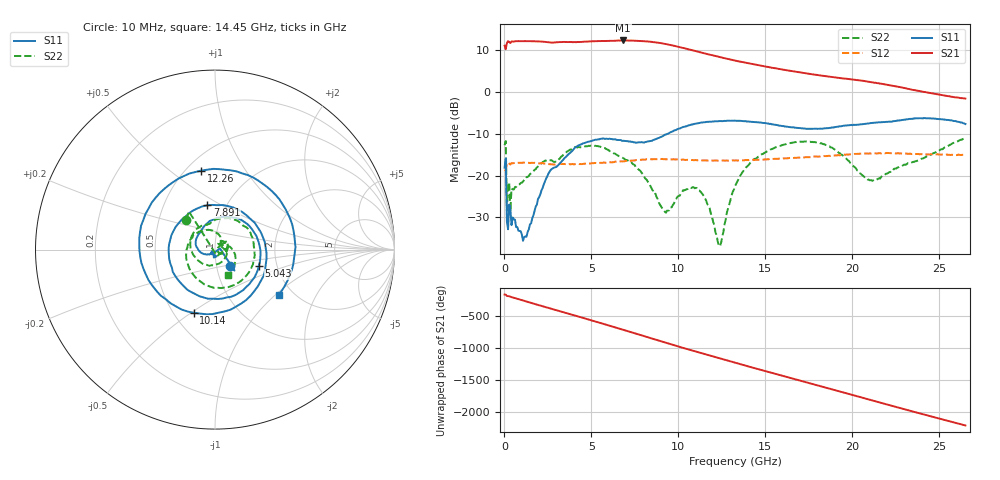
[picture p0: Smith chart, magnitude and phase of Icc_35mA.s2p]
!Keysight Technologies,N5245A,MY52451697,A.10.60.06
!Date: Thursday, May 06, 2021 15:08:13
!Correction: S11(Full 2 Port(1,4))
!S41(Full 2 Port(1,4))
!S14(Full 2 Port(1,4))
!S44(Full 2 Port(1,4))
!S2P File: Measurements: S11, S41, S14, S44:
# Hz S  dB  R 50
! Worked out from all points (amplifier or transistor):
!   401 points, 10 MHz to 26.5 GHz, reference 50 ohm
!   highest |S21| = 12.4 dB at 6.831 GHz (marker M1)
!   |S21| within 3 dB of that: start of sweep to 11.41 GHz
!   unconditionally stable (mu >= 1): start of sweep to end of sweep
!   at 4.381 GHz: K = 1.13, MAG = 12.4 dB, |S12| = -17.3 dB
!   at 13.26 GHz: K = 1.24, MAG = 9.0 dB, |S12| = -16.4 dB
!   at 26.5 GHz: K = 2.55, MAG = -0.2 dB, |S12| = -15.0 dB
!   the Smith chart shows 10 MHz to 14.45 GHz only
!   S11 on the Smith chart (normalised r, x): 10 MHz: 1.16, -0.22; 5.043 GHz: 1.61, -0.32; 7.891 GHz: 0.82, +0.43; 10.14 GHz: 0.63, -0.51; 12.26 GHz: 0.59, +0.65; 14.45 GHz: 1.68, -1.05
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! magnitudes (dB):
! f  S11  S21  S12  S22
! 10 MHz  -18.1  11.1  -18.9  -12.7
! 274.9 MHz  -27.0  12.0  -17.2  -21.7
! 1.136 GHz  -34.7  12.2  -16.9  -21.0
! 2.593 GHz  -19.1  11.9  -17.3  -16.3
! 4.447 GHz  -12.5  12.0  -17.3  -13.3
! 5.043 GHz  -11.7  12.2  -17.0  -12.9
! 6.831 GHz  -11.7  12.4  -16.6  -15.8
! 7.891 GHz  -12.0  12.3  -16.2  -19.4
! 8.884 GHz  -11.0  11.8  -16.1  -26.6
! 9.348 GHz  -10.0  11.5  -16.1  -28.4
! 10.14 GHz  -8.6  10.7  -16.2  -24.3
! 11.33 GHz  -7.3  9.5  -16.4  -24.2
! 11.8 GHz  -7.1  9.0  -16.5  -27.9
! 12.26 GHz  -7.0  8.6  -16.4  -35.8
! 12.46 GHz  -7.0  8.3  -16.4  -36.1
! 13.26 GHz  -6.8  7.6  -16.4  -22.6
! 14.45 GHz  -7.2  6.6  -16.3  -16.0
! 17.69 GHz  -8.8  4.3  -15.5  -11.9
! 18.95 GHz  -8.4  3.5  -15.2  -13.7
! 21 GHz  -7.5  2.4  -14.7  -21.2
! 22.13 GHz  -7.1  1.7  -14.6  -19.2
! 26.5 GHz  -7.6  -1.6  -15.0  -11.1
